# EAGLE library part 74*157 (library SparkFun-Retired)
Quadruple 2-line to 1-line data SELECTOR/MULTIPLEXER RETIRED: IC-09602
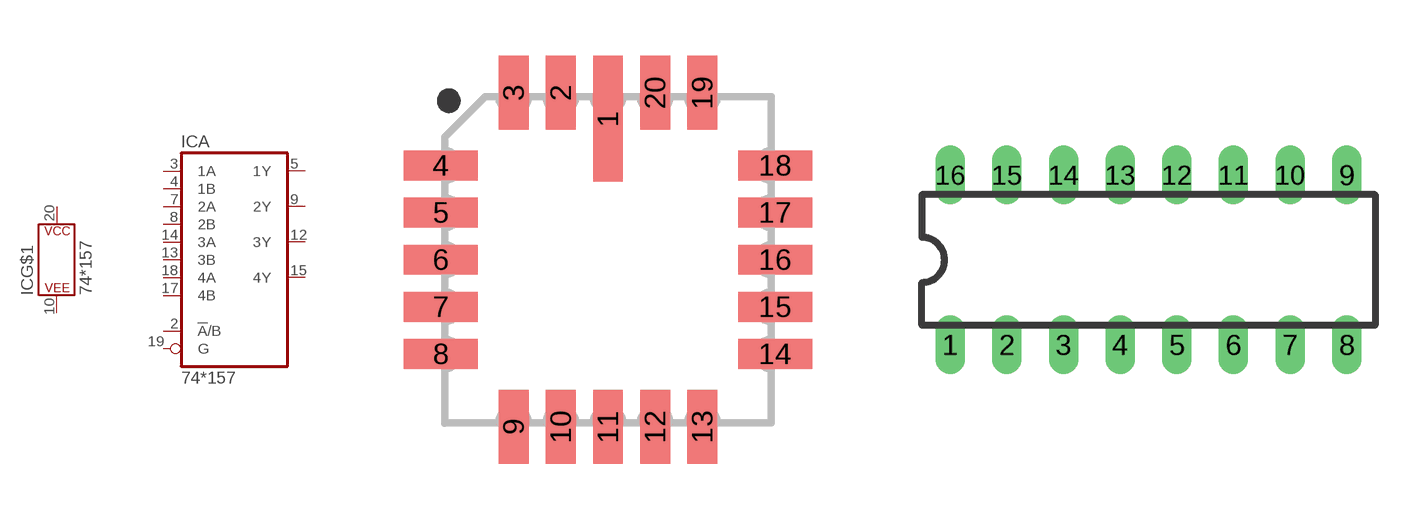
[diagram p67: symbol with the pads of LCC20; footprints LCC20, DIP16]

Designator prefix IC; gates A=74157 G$1=POWER_CONSORT

## 74157FK, 74LS157FK, 74S157FK  [LCC20]
2  A:!A!/B  in
3  A:1A  in
4  A:1B  in
5  A:1Y  out
7  A:2A  in
8  A:2B  in
9  A:2Y  out
10  G$1:P$V-
12  A:3Y  out
13  A:3B  in
14  A:3A  in
15  A:4Y  out
17  A:4B  in
18  A:4A  in
19  A:G  in
20  G$1:P$V+

## 74157N, 74LS157N, 74S157N  [DIP16]
1  A:!A!/B  in
2  A:1A  in
3  A:1B  in
4  A:1Y  out
5  A:2A  in
6  A:2B  in
7  A:2Y  out
8  G$1:P$V-
9  A:3Y  out
10  A:3B  in
11  A:3A  in
12  A:4Y  out
13  A:4B  in
14  A:4A  in
15  A:G  in
16  G$1:P$V+

## 74157SO  [SO16]
Pads as for DIP16

## Footprint LCC20 (pad centres in mm)
Leadless Chip Carrier Ceramic Package
smd 0.8 x 3.4: 1 0,3.8
smd 0.8 x 2: 2 -1.27,4.5; 3 -2.54,4.5; 9 -2.54,-4.5; 10 -1.27,-4.5; 11 0,-4.5; 12 1.27,-4.5; 13 2.54,-4.5; 19 2.54,4.5; 20 1.27,4.5
smd 2 x 0.8: 4 -4.5,2.54; 5 -4.5,1.27; 6 -4.5,0; 7 -4.5,-1.27; 8 -4.5,-2.54; 14 4.5,-2.54; 15 4.5,-1.27; 16 4.5,0; 17 4.5,1.27; 18 4.5,2.54

## Footprint DIP16 (pad centres in mm)
Dual In Line Package
drill 0.813 long: 1 -8.89,-3.81; 2 -6.35,-3.81; 3 -3.81,-3.81; 4 -1.27,-3.81; 5 1.27,-3.81; 6 3.81,-3.81; 7 6.35,-3.81; 8 8.89,-3.81; 9 8.89,3.81; 10 6.35,3.81; 11 3.81,3.81; 12 1.27,3.81; 13 -1.27,3.81; 14 -3.81,3.81; 15 -6.35,3.81; 16 -8.89,3.81

## Footprint SO16 (pad centres in mm)
Small Outline package 150 mil
smd 0.6 x 1.2: 1 -4.445,-2.8; 2 -3.175,-2.8; 3 -1.905,-2.8; 4 -0.635,-2.8; 5 0.635,-2.8; 6 1.905,-2.8; 7 3.175,-2.8; 8 4.445,-2.8; 9 4.445,2.8; 10 3.175,2.8; 11 1.905,2.8; 12 0.635,2.8; 13 -0.635,2.8; 14 -1.905,2.8; 15 -3.175,2.8; 16 -4.445,2.8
